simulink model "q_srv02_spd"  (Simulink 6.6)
settings: Solver=ode1  StartTime=0.0  StopTime=inf  FixedStep=0.002  RelTol=1e-3  AbsTol=1e-6
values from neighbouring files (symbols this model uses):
  a = 10^(-21/20)    (= 0.0891250938134)    [d_lag_q3.m]    (also in d_lead.m = (1+sin(phi_m)) / (1-sin(phi_m)); setup_srv02_exp03_spd.m = 1)
  bsp = 0    [setup_srv02_exp03_spd.m]
  K_AMP = 1    [setup_srv02_exp03_spd.m]    (also in setup_srv02_exp01_mdl.m; setup_srv02_exp02_pos.m)
  K_ENC = 0    [config_srv02.m]
  K_POT = -(352 * pi / 180 / 10)    (= -0.614355896702)    [config_srv02.m]
  K_TACH = -(1000 * 2 * pi / 60 / 1.5 / Kg)    [config_srv02.m]
  Kc = 10^(e_ss_meas/e_ss_min/20)    (= 2.14783047413)    [d_lag_q3.m]    (also in d_lead.m = 53.0884444231; setup_srv02_exp03_spd.m = 0)
  ki = wn^2*tau/K    [d_pi_design.m]    (also in setup_srv02_exp03_spd.m = 0; d_i_design.m = -( -AmpMax + kp * e_ss ) / ti / e_ss; setup_srv02_exp02_pos.m = 0)
  kp = (-1+2*zeta*wn*tau)/K    [d_pi_design.m]    (also in setup_srv02_exp03_spd.m = 0; d_pv_design.m = wn^2/K*tau; setup_srv02_exp02_pos.m = 0)
  T = 10 / (wg_des * a)    [d_lag_q3.m]    (also in d_lead.m = 1 / (w_m * sqrt(a)); setup_srv02_exp03_spd.m = 1)
  VMAX_AMP = 0    [config_srv02.m]
  VMAX_DAC = 10    [setup_srv02_exp03_spd.m]    (also in setup_srv02_exp01_mdl.m; setup_srv02_exp02_pos.m)
  wcf_e = 2 * pi * 63.0    (= 395.840674352)    [setup_srv02_exp03_spd.m]    (also in setup_srv02_exp01_mdl.m = 157.079632679; setup_srv02_exp02_pos.m = 314.159265359)
  zetaf_e = 0.9    [setup_srv02_exp03_spd.m]    (also in setup_srv02_exp01_mdl.m; setup_srv02_exp02_pos.m)
undefined symbols (not defined in the file or in its folder): HIL, qc_get_step_size, square
libraries: quarc_library x5, simulink x3

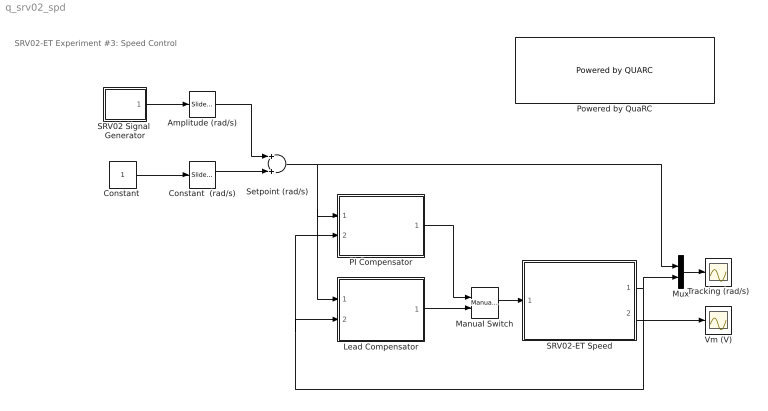
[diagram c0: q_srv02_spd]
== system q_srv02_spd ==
  note: SRV02-ET Experiment #3: Speed Control
  Amplitude (rad/s) : simulink/Math Operations/Slider Gain  SystemSampleTime=-1  low=0  gain=2.5  high=10
  "Constant " : Constant
  Constant  (rad/s) : simulink/Math Operations/Slider Gain  SystemSampleTime=-1  low=-10  gain=5  high=10
  Lead Compensator : Subsystem
  Manual Switch : simulink/Signal Routing/Manual Switch  SystemSampleTime=-1  sw=1  action=0  varsize=off
  Mux : Mux  Inputs=2
  PI Compensator : Subsystem
  Powered by QuaRC : quarc_library/Logos/Powered by QUARC  SystemSampleTime=-1
  SRV02 Signal  Generator : Subsystem  mask(QET Signal Generator){sig_type=square, a=1, f=0.4}
      mask prompts: sig_type "Signal Type"; a "Amplitude"; f "Frequency (Hz)"
      mask help: Generates a square, triangular, or sinusoidal waveform of a specified amplitude and frequency.
  SRV02-ET Speed : Subsystem
  Setpoint (rad/s) : Sum  OutScaling=2^-10
  Tracking (rad/s) : Scope
  Vm (V) : Scope
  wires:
  Setpoint (rad/s)/1 -> PI Compensator/1(wd (rad/s)), Lead Compensator/1(wd (rad/s)), Mux/1
  SRV02-ET Speed/2(Vm (V)) -> Vm (V)/1
  Mux/1 -> Tracking (rad/s)/1
  SRV02 Signal  Generator/1(out) -> Amplitude (rad/s)/1
  Amplitude (rad/s)/1 -> Setpoint (rad/s)/1
  "Constant "/1 -> Constant  (rad/s)/1
  SRV02-ET Speed/1(omega_l (rad/s)) -> PI Compensator/2(wl (rad/s)), Lead Compensator/2(wl (rad/s)), Mux/2
  PI Compensator/1(Vi (V)) -> Manual Switch/1
  Lead Compensator/1(Vi (V)) -> Manual Switch/2
  Manual Switch/1 -> SRV02-ET Speed/1(Vi (V))
  Constant  (rad/s)/1 -> Setpoint (rad/s)/2

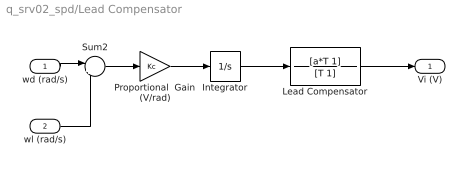
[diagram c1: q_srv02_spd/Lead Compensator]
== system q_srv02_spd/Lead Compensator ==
  wd (rad/s) : Inport
  wl (rad/s) : Inport  Port=2
  Integrator : Integrator
  Lead Compensator : TransferFcn  Numerator=[a*T 1]  Denominator=[T 1]
  Proportional  Gain (V/rad) : Gain  Gain=Kc
  Sum2 : Sum  Inputs=|+-
  Vi (V) : Outport
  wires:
  wl (rad/s)/1 -> Sum2/2
  wd (rad/s)/1 -> Sum2/1
  Lead Compensator/1 -> Vi (V)/1
  Sum2/1 -> Proportional  Gain (V/rad)/1
  Proportional  Gain (V/rad)/1 -> Integrator/1
  Integrator/1 -> Lead Compensator/1

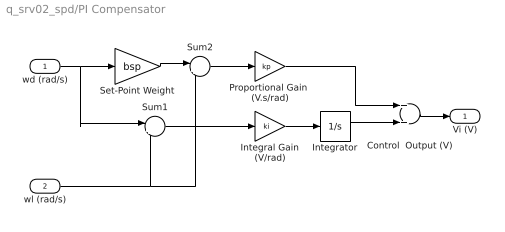
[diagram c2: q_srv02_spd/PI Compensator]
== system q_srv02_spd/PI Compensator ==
  wd (rad/s) : Inport
  wl (rad/s) : Inport  Port=2
  Control  Output (V) : Sum  OutScaling=2^-10
  Integral Gain (V/rad) : Gain  Gain=ki
  Integrator : Integrator  UpperSaturationLimit=10  LowerSaturationLimit=-10
  Proportional Gain  (V.s/rad) : Gain  Gain=kp
  Set-Point Weight : Gain  Gain=bsp
  Sum1 : Sum  Inputs=|+-
  Sum2 : Sum  Inputs=|+-
  Vi (V) : Outport
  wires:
  wl (rad/s)/1 -> Sum2/2, Sum1/2
  Control  Output (V)/1 -> Vi (V)/1
  wd (rad/s)/1 -> Sum1/1, Set-Point Weight/1
  Sum2/1 -> Proportional Gain  (V.s/rad)/1
  Set-Point Weight/1 -> Sum2/1
  Proportional Gain  (V.s/rad)/1 -> Control  Output (V)/1
  Integrator/1 -> Control  Output (V)/2
  Integral Gain (V/rad)/1 -> Integrator/1
  Sum1/1 -> Integral Gain (V/rad)/1

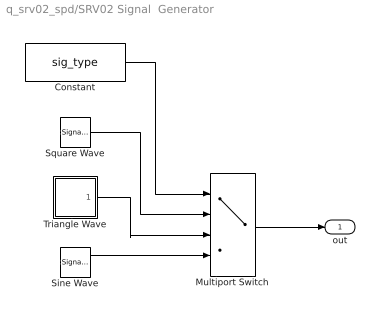
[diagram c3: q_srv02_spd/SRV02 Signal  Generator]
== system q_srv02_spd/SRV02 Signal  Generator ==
  Constant : Constant  Value=sig_type
  Multiport Switch : MultiPortSwitch  Inputs=3
  Sine Wave : SignalGenerator  Amplitude=a  Frequency=f
  Square Wave : SignalGenerator  WaveForm=square  Amplitude=a  Frequency=f
  Triangle Wave : Subsystem
  out : Outport
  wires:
  Constant/1 -> Multiport Switch/1
  Multiport Switch/1 -> out/1
  Sine Wave/1 -> Multiport Switch/4
  Triangle Wave/1(out) -> Multiport Switch/3
  Square Wave/1 -> Multiport Switch/2

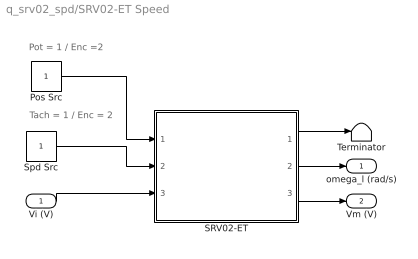
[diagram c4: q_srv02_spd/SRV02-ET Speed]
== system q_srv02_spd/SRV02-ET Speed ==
  note: Pot = 1 / Enc =2
  note: Tach = 1 / Enc = 2
  Vi (V) : Inport
  Pos Src : Constant
  SRV02-ET : Subsystem
  Spd Src : Constant
  Terminator : Terminator
  omega_l (rad/s) : Outport
  Vm (V) : Outport  Port=2
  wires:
  Pos Src/1 -> SRV02-ET/1(pos src)
  SRV02-ET/1(theta_l (rad)) -> Terminator/1
  Spd Src/1 -> SRV02-ET/2(spd src)
  Vi (V)/1 -> SRV02-ET/3(Vi (V))
  SRV02-ET/3(Vm (V)) -> Vm (V)/1
  SRV02-ET/2(omega_l (rad/s)) -> omega_l (rad/s)/1

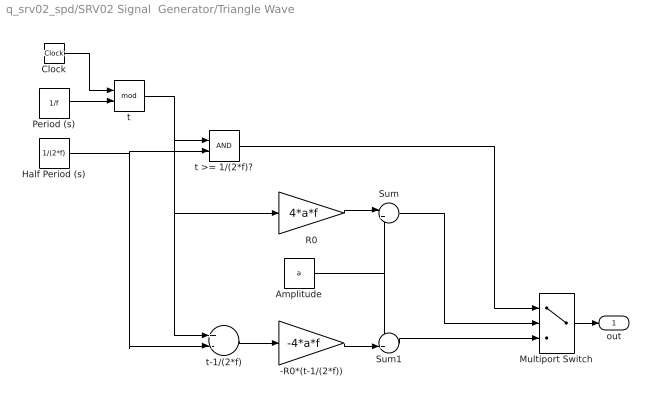
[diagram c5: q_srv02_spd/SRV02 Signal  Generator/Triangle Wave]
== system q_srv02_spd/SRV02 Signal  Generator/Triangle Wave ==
  -R0*(t-1/(2*f)) : Gain  Gain=-4*a*f
  Amplitude : Constant  Value=a
  Clock : Clock
  Half Period (s) : Constant  Value=1/(2*f)
  Multiport Switch : MultiPortSwitch  Inputs=2  zeroidx=on
  Period (s) : Constant  Value=1/f
  R0 : Gain  Gain=4*a*f
  Sum : Sum  Inputs=|+-
  Sum1 : Sum  Inputs=++|
  t : Math  Operator=mod
  t >= 1/(2*f)? : RelationalOperator  LogicOutDataTypeMode=Boolean
  t-1/(2*f) : Sum  Inputs=+-  OutScaling=2^-10
  out : Outport
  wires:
  Multiport Switch/1 -> out/1
  Clock/1 -> t/1
  Period (s)/1 -> t/2
  t/1 -> t >= 1/(2*f)?/1, R0/1, t-1/(2*f)/1
  Half Period (s)/1 -> t >= 1/(2*f)?/2, t-1/(2*f)/2
  t-1/(2*f)/1 -> -R0*(t-1/(2*f))/1
  R0/1 -> Sum/1
  Amplitude/1 -> Sum/2, Sum1/1
  -R0*(t-1/(2*f))/1 -> Sum1/2
  t >= 1/(2*f)?/1 -> Multiport Switch/1
  Sum/1 -> Multiport Switch/2
  Sum1/1 -> Multiport Switch/3

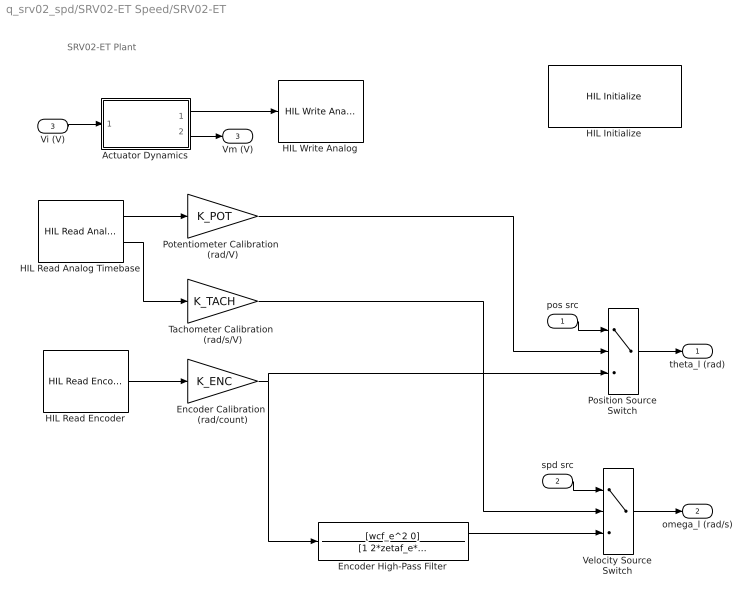
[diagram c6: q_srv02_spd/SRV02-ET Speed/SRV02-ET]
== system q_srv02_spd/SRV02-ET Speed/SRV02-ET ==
  note: SRV02-ET Plant
  pos src : Inport
  spd src : Inport  Port=2
  Vi (V) : Inport  Port=3
  Actuator Dynamics : Subsystem
  Encoder Calibration  (rad/count) : Gain  Gain=K_ENC
  Encoder High-Pass Filter : TransferFcn  Numerator=[wcf_e^2 0]  Denominator=[1 2*zetaf_e*wcf_e wcf_e^2]
  HIL Initialize : quarc_library/Data Acquisition/Generic/Configuration/HIL Initialize  object_name=HIL-1  board_type=q8  board_number=0  exclusive=off  active=on  hardware_clocks=0:1  clock_modes=[0 0]  set_clock_params_at_start=on  set_clock_params_at_switch_in=off  analog_input_channels=0:7  analog_input_maximums=10  analog_input_minimums=-10  set_analog_input_params_at_start=on  set_analog_input_params_at_switch_in=off  analog_output_channels=0:7  analog_output_maximums=10  analog_output_minimums=-10  initial_analog_outputs=0  final_analog_outputs=0  watchdog_analog_outputs=0  set_analog_output_params_at_start=on  set_analog_output_params_at_switch_in=off  set_analog_outputs_at_start=on  set_analog_outputs_at_switch_in=off  set_analog_outputs_at_terminate=on  set_analog_outputs_at_switch_out=off  set_analog_outputs_on_watchdog=off  digital_input_channels=[]  digital_output_channels=[]  digital_output_configuration=[]  initial_digital_outputs=1  final_digital_outputs=1  watchdog_digital_outputs=0  set_digital_output_params_at_start=off  set_digital_output_params_at_switch_in=off  set_digital_outputs_at_start=on  set_digital_outputs_at_switch_in=off  set_digital_outputs_at_terminate=on  set_digital_outputs_at_switch_out=off  set_digital_outputs_on_watchdog=off  encoder_channels=0:7  quadrature=4  encoder_filter_frequency=(1/120e-9)/1  initial_encoder_counts=0  set_encoder_params_at_start=on  set_encoder_params_at_switch_in=off  set_encoder_counts_at_start=on  set_encoder_counts_at_switch_in=off  pwm_channels=[]  pwm_modes=0  pwm_frequency=(1/60e-9)/1024  pwm_configuration=[]  pwm_alignment=[]  pwm_polarity=[]  pwm_leading_deadband=[]  pwm_trailing_deadband=[]  initial_pwm_outputs=0  final_pwm_outputs=0  watchdog_pwm_outputs=0  set_pwm_params_at_start=on  set_pwm_params_at_switch_in=off  set_pwm_outputs_at_start=on  set_pwm_outputs_at_switch_in=off  set_pwm_outputs_at_terminate=on  set_pwm_outputs_at_switch_out=off  set_pwm_outputs_on_watchdog=off  other_output_channels=[]  initial_other_outputs=[]  final_other_outputs=[]  watchdog_other_outputs=0  set_other_outputs_at_start=on  set_other_outputs_at_switch_in=off  set_other_outputs_at_terminate=on  set_other_outputs_at_switch_out=off  set_other_outputs_on_watchdog=off
  HIL Read Analog Timebase : quarc_library/Data Acquisition/Generic/Timebases/HIL Read Analog Timebase  Tag=unassigned  object_name=HIL-1  clock=0  channels=[0,1]  samples_in_buffer=max(ceil(1/qc_get_step_size), 1)  active=on  vector_output=off
  HIL Read Encoder : quarc_library/Data Acquisition/Generic/Immediate I//O/HIL Read Encoder  Tag=unassigned  object_name=HIL-1  channels=0  sample_time=qc_get_step_size  active=on  vector_output=off  data_type_mode=Inherit via back propagation  data_type=double
  HIL Write Analog : quarc_library/Data Acquisition/Generic/Immediate I//O/HIL Write Analog  Tag=unassigned  object_name=HIL-1  channels=0  sample_time=-1  active=off  vector_input=off
  Position Source Switch : MultiPortSwitch  Inputs=2
  Potentiometer Calibration  (rad/V) : Gain  Gain=K_POT
  Tachometer Calibration  (rad/s/V) : Gain  Gain=K_TACH
  Velocity Source Switch : MultiPortSwitch  Inputs=2
  theta_l (rad) : Outport  InitialOutput=0
  omega_l (rad/s) : Outport  Port=2  InitialOutput=0
  Vm (V) : Outport  Port=3  InitialOutput=0
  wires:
  HIL Read Analog Timebase/2 -> Tachometer Calibration  (rad/s/V)/1
  HIL Read Encoder/1 -> Encoder Calibration  (rad/count)/1
  Encoder High-Pass Filter/1 -> Velocity Source Switch/3
  Potentiometer Calibration  (rad/V)/1 -> Position Source Switch/2
  spd src/1 -> Velocity Source Switch/1
  pos src/1 -> Position Source Switch/1
  Position Source Switch/1 -> theta_l (rad)/1
  Velocity Source Switch/1 -> omega_l (rad/s)/1
  Actuator Dynamics/2(Vm (V)) -> Vm (V)/1
  Actuator Dynamics/1(Vdaq (V)) -> HIL Write Analog/1
  HIL Read Analog Timebase/1 -> Potentiometer Calibration  (rad/V)/1
  Vi (V)/1 -> Actuator Dynamics/1(Vi (V))
  Encoder Calibration  (rad/count)/1 -> Position Source Switch/3, Encoder High-Pass Filter/1
  Tachometer Calibration  (rad/s/V)/1 -> Velocity Source Switch/2

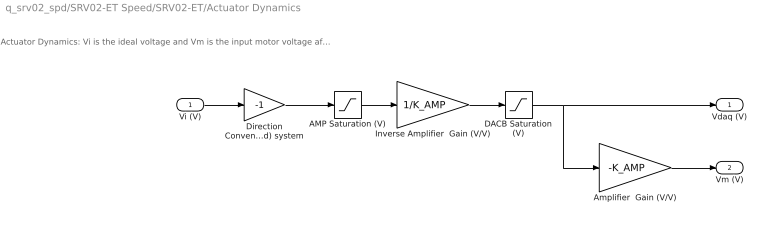
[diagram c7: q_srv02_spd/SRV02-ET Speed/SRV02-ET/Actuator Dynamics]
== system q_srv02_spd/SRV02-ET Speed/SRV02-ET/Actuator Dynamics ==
  note: Actuator Dynamics: Vi is the ideal voltage and Vm is the input motor voltage after going through the DACB and amplifier limitiations.
  Vi (V) : Inport
  AMP Saturation (V) : Saturate  UpperLimit=VMAX_AMP  LowerLimit=-VMAX_AMP
  Amplifier  Gain (V/V) : Gain  Gain=-K_AMP
  DACB Saturation (V) : Saturate  UpperLimit=VMAX_DAC  LowerLimit=-VMAX_DAC
  Direction Convention: (Right-Hand) system : Gain  Gain=-1
  Inverse Amplifier  Gain (V/V) : Gain  Gain=1/K_AMP
  Vdaq (V) : Outport
  Vm (V) : Outport  Port=2
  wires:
  Direction Convention: (Right-Hand) system/1 -> AMP Saturation (V)/1
  Amplifier  Gain (V/V)/1 -> Vm (V)/1
  DACB Saturation (V)/1 -> Vdaq (V)/1, Amplifier  Gain (V/V)/1
  Inverse Amplifier  Gain (V/V)/1 -> DACB Saturation (V)/1
  AMP Saturation (V)/1 -> Inverse Amplifier  Gain (V/V)/1
  Vi (V)/1 -> Direction Convention: (Right-Hand) system/1
